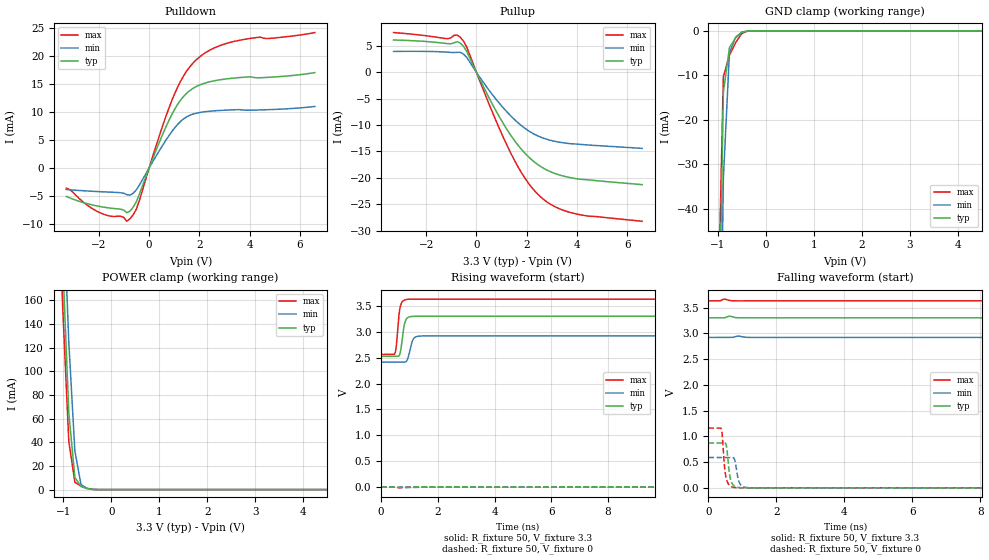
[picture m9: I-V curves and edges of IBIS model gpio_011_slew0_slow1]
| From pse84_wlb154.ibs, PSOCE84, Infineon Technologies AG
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[Model] gpio_011_slew0_slow1
Model_type I/O
Enable   Active-High
Vinl  =  0.99
Vinh  =  2.31
Vmeas =  1.65
Cref  =  15e-12
| Capacitance   typ   min   max
C_comp   1.09946e-12   1.08623e-12   1.11440e-12
| Variables   typ   min   max
[GND Clamp Reference]   0   0   0
[POWER Clamp Reference]   3.3   2.92   3.63
[Pulldown Reference]   0   0   0
[Pullup Reference]   3.3   2.92   3.63
[Temperature Range]   25   125   -40
[Voltage Range]   3.3   2.92   3.63
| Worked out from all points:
|   slope of the pulldown table from 0 to 0.495 V, typ, clamps not added: 89.5 ohm
|   slope of the pullup table from 0 to 0.495 V, typ, clamps not added: 104 ohm
|   GND clamp passes 1 mA (typ) near -0.57 V on its own axis
|   POWER clamp passes 1 mA (typ) near -0.52 V on its own axis
|   falling waveform, R_fixture 50, V_fixture 3.3: 20-80 % time 572ns typ, 878ns min, 316ns max; typ from 3.3 V to 2.52 V
|   falling waveform, R_fixture 50, V_fixture 0: 20-80 % time 95.3ps typ, 104ps min, 91.7ps max; typ from 0.871 V to 0 V
|   rising waveform, R_fixture 50, V_fixture 3.3: 20-80 % time 120ps typ, 143ps min, 107ps max; typ from 2.52 V to 3.3 V
|   rising waveform, R_fixture 50, V_fixture 0: 20-80 % time 563ns typ, 850ns min, 340ns max; typ from 0 V to 0.871 V
[GND Clamp]
| Voltage   I(typ)   I(min)   I(max)
-1.65V    -892.5mA   -911.9mA   -883.9mA
-1.015V   -92.32mA   -129.7mA   -71.28mA
-888.3mV  -13.83mA   -33.21mA   -10.31mA
-761.4mV  -3.792mA   -4.944mA   -5.509mA
-634.5mV  -1.622mA   -1.436mA   -2.707mA
-507.6mV  -326.2uA   -352.3uA   -651.6uA
-380.7mV  -13.48uA   -32.14uA   -19.55uA
-253.8mV  -189.4nA   -1.276uA   -466.7nA
6.6V      0A         0A         0A
[POWER Clamp]
| Voltage   I(typ)   I(min)   I(max)
-1.523V   838.1mA    872.9mA    823.9mA
-1.142V   346.5mA    405.1mA    310.5mA
-1.015V   193mA      257.4mA    153.9mA
-888.3mV  64.97mA    124.9mA    40.96mA
-761.4mV  10.28mA    32.7mA     6.184mA
-634.5mV  2.553mA    4.346mA    3.067mA
-507.6mV  805.9uA    960.7uA    1.159mA
-253.8mV  1.454uA    10.02uA    1.678uA
6.6V      0A         0A         0A
[Pulldown]
| Voltage   I(typ)   I(min)   I(max)
-3.3V     -5.082mA   -3.847mA   -3.58mA
-2.157V   -6.699mA   -4.185mA   -7.533mA
-1.142V   -7.349mA   -4.412mA   -8.601mA
-888.3mV  -7.984mA   -4.764mA   -9.517mA
-507.6mV  -6.006mA   -3.898mA   -7.337mA
341.4mV   3.871mA    2.599mA    4.846mA
910.3mV   9.579mA    6.524mA    12.1mA
1.366V    12.74mA    8.739mA    16.39mA
1.821V    14.4mA     9.707mA    19.05mA
2.503V    15.47mA    10.16mA    21.23mA
3.3V      16.01mA    10.37mA    22.49mA
6.6V      17.02mA    10.98mA    24.16mA
[Pullup]
| Voltage   I(typ)   I(min)   I(max)
-3.3V     6.119mA    3.957mA    7.53mA
-1.142V   5.434mA    3.812mA    6.371mA
-761.4mV  5.81mA     3.793mA    7.069mA
-634.5mV  5.494mA    3.779mA    6.598mA
-380.7mV  3.894mA    2.777mA    4.724mA
682.8mV   -6.455mA   -4.515mA   -8.084mA
1.479V    -12.69mA   -8.783mA   -16.35mA
2.048V    -15.9mA    -11mA      -20.85mA
2.731V    -18.33mA   -12.58mA   -24.29mA
3.3V      -19.44mA   -13.24mA   -25.84mA
4.051V    -20.21mA   -13.62mA   -26.91mA
6.6V      -21.29mA   -14.41mA   -28.23mA
[Ramp]
dV/dt_r   0.522554/0.563283u  0.352068/0.8504u  0.696443/0.340427u
dV/dt_f   0.464761/0.572062u  0.302569/0.878256u  0.64065/0.315805u
R_load = 50
[Falling Waveform]
R_fixture = 50
V_fixture = 3.3
V_fixture_min = 2.92
V_fixture_max = 3.63
| Time   V(typ)   V(min)   V(max)
0s        3.3V       2.92V      3.63V
111.3ns   3.3V       2.92V      3.606V
181ns     3.296V     2.92V      3.389V
279.8ns   3.207V     2.917V     3.097V
402ns     3.044V     2.885V     2.872V
564.9ns   2.873V     2.798V     2.718V
768.5ns   2.737V     2.695V     2.632V
1.172us   2.607V     2.562V     2.579V
1.797us   2.546V     2.47V      2.564V
4us       2.525V     2.416V     2.562V
[Falling Waveform]
R_fixture = 50
V_fixture = 0
V_fixture_min = 0
V_fixture_max = 0
| Time   V(typ)   V(min)   V(max)
0s        871.4mV    589.6mV    1.161V
379.2ps   871.3mV    589.5mV    1.145V
504ps     866mV      589.6mV    254mV
542.9ps   756.1mV    589.6mV    141.9mV
619.3ps   271.9mV    589.7mV    48.77mV
670.2ps   125.6mV    589.8mV    23.85mV
768.1ps   33.6mV     554.6mV    6.148mV
876.7ps   8.22mV     170.9mV    1.057mV
952ps     2.957mV    57.88mV    472.6uV
4us       19.29nV    580nV      11.01nV
[Rising Waveform]
R_fixture = 50
V_fixture = 3.3
V_fixture_min = 2.92
V_fixture_max = 3.63
| Time   V(typ)   V(min)   V(max)
0s        2.525V     2.414V     2.562V
480.8ps   2.525V     2.414V     2.576V
539.3ps   2.525V     2.413V     2.747V
636.3ps   2.54V      2.414V     3.355V
698.9ps   2.669V     2.414V     3.528V
792.6ps   3.059V     2.413V     3.604V
857.5ps   3.211V     2.417V     3.619V
940.6ps   3.273V     2.483V     3.627V
1.139ns   3.298V     2.86V      3.629V
4us       3.3V       2.92V      3.63V
[Rising Waveform]
R_fixture = 50
V_fixture = 0
V_fixture_min = 0
V_fixture_max = 0
| Time   V(typ)   V(min)   V(max)
0s        19.02nV    575.2nV    11.35nV
113.3ns   151.3uV    103.6uV    33.68mV
197.6ns   23.45mV    826.8uV    263.4mV
305.9ns   143.2mV    16.78mV    571.8mV
450.6ns   336.5mV    80.85mV    843.3mV
613.5ns   514.6mV    175.6mV    992.6mV
817.1ns   660.6mV    286.3mV    1.076V
1.193us   784.2mV    428.7mV    1.134V
1.796us   845.6mV    529.6mV    1.156V
4us       870.9mV    586.8mV    1.161V
